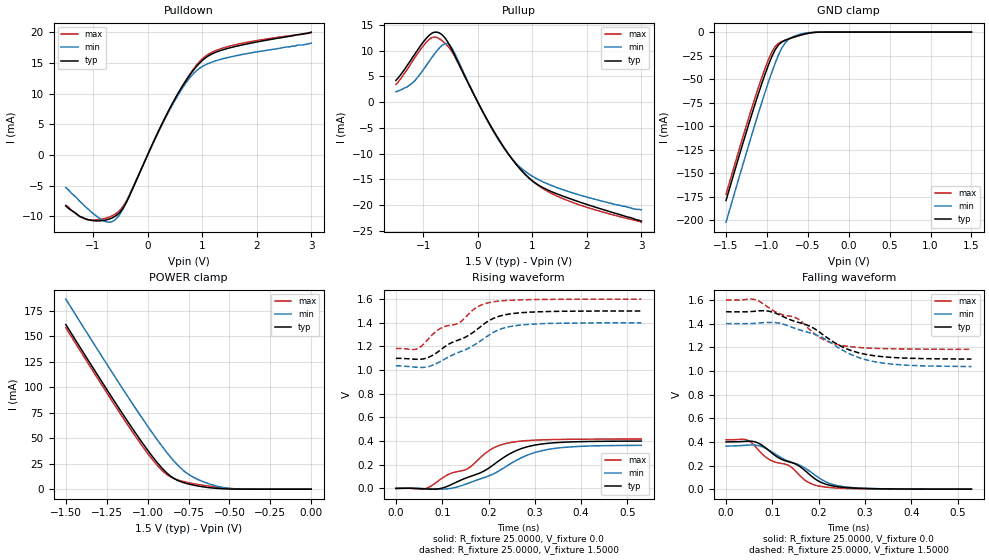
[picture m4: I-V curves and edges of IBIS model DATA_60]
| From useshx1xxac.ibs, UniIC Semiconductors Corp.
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|   Model DATA_60
[Model]  DATA_60
Model_type   I/O
Polarity   Non-Inverting
Enable   Active-High
Vinl =   0.600000V
Vinh =   0.900000V
Vmeas =   0.750000V
Rref =   25.000000
Vref =   0.7500000V
C_comp   1.3900pF   1.3640pF   1.5600pF
[Temperature Range]   25.0000   95.0000   0.0
[Voltage Range]   1.5000V   1.4000V   1.6000V
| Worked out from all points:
|   slope of the pulldown table from 0 to 0.225 V, typ, clamps not added: 51.6 ohm
|   slope of the pullup table from 0 to 0.225 V, typ, clamps not added: 51.1 ohm
|   GND clamp passes 1 mA (typ) near -0.48 V on its own axis
|   POWER clamp passes 1 mA (typ) near -0.59 V on its own axis
|   rising waveform, R_fixture 25.0000, V_fixture 0.0: 20-80 % time 114ps typ, 114ps min, 108ps max; typ from 0 V to 0.4 V
|   rising waveform, R_fixture 25.0000, V_fixture 1.5000: 20-80 % time 103ps typ, 102ps min, 98.6ps max; typ from 1.1 V to 1.5 V
|   falling waveform, R_fixture 25.0000, V_fixture 0.0: 20-80 % time 100ps typ, 101ps min, 98.8ps max; typ from 0.4 V to 0 V
|   falling waveform, R_fixture 25.0000, V_fixture 1.5000: 20-80 % time 117ps typ, 114ps min, 111ps max; typ from 1.5 V to 1.1 V
[Pulldown]
|Voltage   I(typ)   I(min)   I(max)
-1.5V     -8.3mA     -5.3mA     -8.2mA
-1.1V     -10.51mA   -8.75mA    -10.54mA
-800mV    -10.65mA   -10.74mA   -10.36mA
-600mV    -10.01mA   -10.6mA    -9.663mA
-400mV    -7.919mA   -7.889mA   -7.652mA
100mV     1.987mA    1.924mA    1.931mA
450mV     8.306mA    8.07mA     8.208mA
700mV     12.06mA    11.68mA    12.1mA
900mV     14.44mA    13.74mA    14.67mA
1.1V      16.05mA    14.83mA    16.31mA
1.45V     17.3mA     15.81mA    17.59mA
3V        20mA       18.2mA     19.9mA
[Pullup]
|Voltage   I(typ)   I(min)   I(max)
-1.5V     4.2mA      2mA        3.4mA
-1.15V    9.36mA     4.18mA     8.68mA
-850mV    13.3mA     8.51mA     12.46mA
-700mV    13.39mA    10.53mA    12.28mA
-550mV    11.67mA    11.36mA    10.87mA
-450mV    9.677mA    10.06mA    9.384mA
300mV     -5.771mA   -5.921mA   -5.749mA
550mV     -9.892mA   -9.938mA   -9.875mA
800mV     -13.24mA   -12.85mA   -13.26mA
1.1V      -16.02mA   -14.96mA   -16.12mA
1.55V     -18.2mA    -16.96mA   -18.68mA
3V        -23.1mA    -20.9mA    -23.3mA
[GND_clamp]
|Voltage   I(typ)   I(min)   I(max)
-1.5V     -178.7mA   -201.8mA   -172.1mA
-1.18V    -85.9mA    -107.5mA   -79.02mA
-1.06V    -53.85mA   -73.82mA   -47.38mA
-980mV    -34.46mA   -52.52mA   -28.79mA
-940mV    -25.94mA   -42.47mA   -21.09mA
-900mV    -18.8mA    -33.04mA   -15.34mA
-860mV    -13.68mA   -24.5mA    -11.91mA
-780mV    -8.804mA   -11.75mA   -8.617mA
-740mV    -7.413mA   -8.071mA   -7.384mA
-620mV    -3.934mA   -2.917mA   -4.046mA
-420mV    -302.4uA   -187.9uA   -428.5uA
1.5V      1.623nA    17.64nA    1.98nA
[POWER_clamp]
|Voltage   I(typ)   I(min)   I(max)
-1.5V     161.3mA    186.3mA    158.3mA
-1.22V    90.37mA    115.2mA    87.1mA
-1.04V    47.2mA     71.18mA    43.94mA
-980mV    33.96mA    57.17mA    30.91mA
-920mV    22.07mA    43.79mA    19.67mA
-880mV    15.49mA    35.42mA    14.07mA
-840mV    10.61mA    27.72mA    10.46mA
-780mV    6.409mA    18.15mA    7.405mA
-720mV    3.991mA    11.66mA    5.381mA
-560mV    586.1uA    2.318mA    1.645mA
-440mV    47uA       184.9uA    218uA
0V        1.623nA    5.301nA    2.263nA
[Ramp]
| variable   typ   min   max
dV/dt_r  0.2403/0.1158n   0.2188/0.1157n   0.2506/0.1097n
dV/dt_f  0.2406/0.1185n   0.2184/0.1147n   0.2508/0.1114n
R_load = 25.0000
[Rising Waveform]
R_fixture= 25.0000
V_fixture= 0.0
V_fixture_min= 0.0
V_fixture_max= 0.0
|time   V(typ)   V(min)   V(max)
0s        0V         0V         0V
65ps      -4.494mV   -2.796mV   -88.05uV
105ps     8.716mV    -5.447mV   99.82mV
155ps     93.27mV    42mV       167mV
185ps     136.6mV    83.91mV    269.9mV
205ps     183.7mV    112.7mV    329.3mV
245ps     290.5mV    202.6mV    386.1mV
290ps     357.8mV    290.2mV    405.7mV
340ps     385mV      336.4mV    412.8mV
530ps     399.8mV    363.7mV    417.3mV
[Rising Waveform]
R_fixture= 25.0000
V_fixture= 1.5000
V_fixture_min= 1.4000
V_fixture_max= 1.6000
|time   V(typ)   V(min)   V(max)
0s        1.099V     1.036V     1.182V
45ps      1.091V     1.024V     1.179V
70ps      1.107V     1.029V     1.263V
95ps      1.166V     1.07V      1.349V
135ps     1.254V     1.149V     1.396V
175ps     1.343V     1.226V     1.532V
210ps     1.436V     1.318V     1.577V
235ps     1.467V     1.358V     1.587V
285ps     1.489V     1.386V     1.595V
530ps     1.5V       1.4V       1.6V
[Falling Waveform]
R_fixture= 25.0000
V_fixture= 0.0
V_fixture_min= 0.0
V_fixture_max= 0.0
|time   V(typ)   V(min)   V(max)
0s        399.8mV    363.7mV    417.3mV
45ps      405.2mV    371.8mV    416.1mV
65ps      397.1mV    371.5mV    353.3mV
90ps      334.7mV    335.7mV    258.9mV
135ps     231.8mV    236.7mV    201.2mV
170ps     158.9mV    179.4mV    77.27mV
200ps     67.86mV    97.31mV    26.97mV
230ps     27.88mV    40.35mV    12.02mV
275ps     9.502mV    12.76mV    4.718mV
530ps     0V         0V         0V
[Falling Waveform]
R_fixture= 25.0000
V_fixture= 1.5000
V_fixture_min= 1.4000
V_fixture_max= 1.6000
|time   V(typ)   V(min)   V(max)
0s        1.5V       1.4V       1.6V
60ps      1.503V     1.401V     1.605V
100ps     1.497V     1.409V     1.514V
155ps     1.411V     1.351V     1.44V
195ps     1.346V     1.304V     1.302V
220ps     1.276V     1.253V     1.247V
255ps     1.196V     1.168V     1.211V
290ps     1.149V     1.108V     1.197V
340ps     1.119V     1.065V     1.188V
530ps     1.099V     1.036V     1.182V
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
